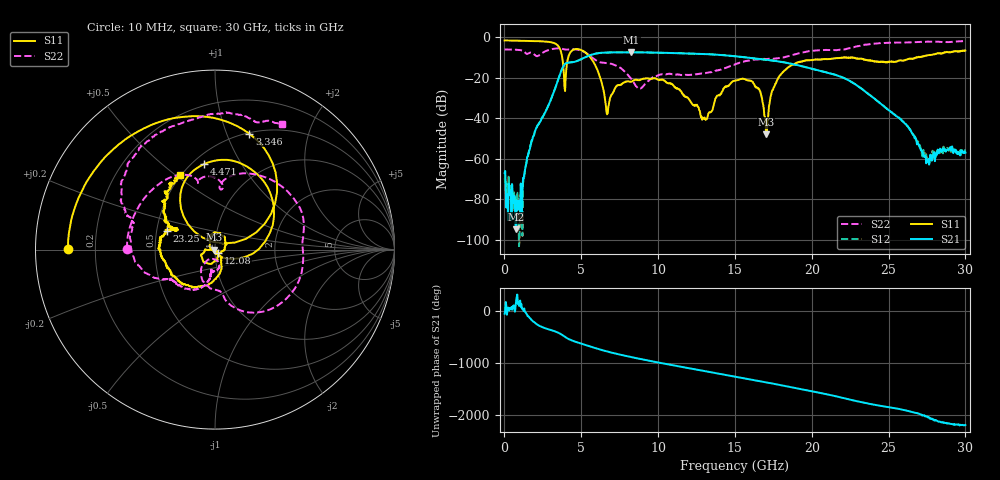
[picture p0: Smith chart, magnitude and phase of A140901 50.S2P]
!  2-Port S-parameters saved by WinCal
! VAR MeasName=S-Parameters (CALIBRATED_DATA) read from VNA (N5244A)
! VAR MeasDate=11/3/2014 9:35:49 AM
! VAR NAME=A140901 50
! VAR FILENAME=A140901 50.S2P
! VAR DATE=11/3/2014 9:35:50 AM
! VAR PHYS_PORTS=1,2
# Hz S RI R 50
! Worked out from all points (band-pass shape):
!   801 points, 10 MHz to 30 GHz, reference 50 ohm
!   highest |S21| = -7.53 dB at 8.257 GHz (marker M1); lowest = -94.8 dB at 759.8 MHz (marker M2)
!   |S21| within 3 dB of the highest: 5.107 GHz to 16.22 GHz (11.11 GHz wide, 104 % of centre)
!   lowest |S11| = -47.9 dB at 17.03 GHz (marker M3), VSWR 1.01, Z = 49.6 - j0.0285 ohm
!   |S11| at or under -10 dB: 3.756 GHz to 4.154 GHz (397.9 MHz wide, 10.1 % of centre); 5.58 GHz to 22.08 GHz (16.5 GHz wide, 119 % of centre); 22.1 GHz to 26.84 GHz (4.749 GHz wide, 19.4 % of centre)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
!   |S22| runs from -25.5 to -2.0 dB; largest |S21 - S12| = 0.0029
!   S11 on the Smith chart (normalised r, x): 10 MHz: 0.10, +0.00; 3.346 GHz: 0.51, +1.21; 4.471 GHz: 0.57, +0.70; 12.08 GHz: 1.03, -0.04; 23.25 GHz: 0.57, +0.13; 30 GHz: 0.49, +0.52
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1e7  -0.8175 0.00333  0.000247 -0.000369  0.000278 -0.000174  -0.4911 0.00373
7.5975e8  -0.7772 0.2442  -1.81e-05 -2.44e-06  2.49e-05 -3.71e-05  -0.3671 0.3175
1.921862e9  -0.5489 0.5745  -0.00304 0.00218  -0.00298 0.00225  0.0354 0.3725
3.346388e9  0.1907 0.6461  0.0441 -0.0413  0.0445 -0.0414  0.4163 0.3111
3.946188e9  -0.0154 0.0438  -0.1737 -0.13  -0.174 -0.1296  0.4878 0.0504
4.471012e9  -0.0615 0.4764  -0.1818 0.1566  -0.181 0.1564  0.4791 -0.1403
5.033325e9  0.2665 0.3866  0.0283 0.2868  0.0282 0.2863  0.3113 -0.3316
5.970512e9  0.1769 -0.0378  0.3899 -0.025  0.3897 -0.0242  0.048 -0.2599
6.682775e9  -0.00831 -0.00921  0.1857 -0.37  0.1858 -0.3693  0.00449 -0.2241
8.25725e9  -0.0194 0.0766  -0.4159 -0.0597  -0.4144 -0.0602  -0.0561 -0.0736
1.001916e10  0.0384 0.0793  0.0471 0.408  0.0469 0.4069  0.0118 -0.1132
1.208098e10  0.0165 -0.0209  0.3392 -0.194  0.3389 -0.1933  -0.0218 -0.1142
1.305565e10  -0.0016 -0.00934  0.0515 -0.3763  0.0504 -0.3754  -0.0247 -0.1251
1.5005e10  -0.0264 -0.0789  -0.3307 0.0491  -0.3299 0.0498  -0.0607 -0.2027
1.65045e10  -0.0529 -0.000149  -0.00313 0.2881  -0.00347 0.2885  -0.1895 -0.2063
1.702932e10  -0.00403 -0.000287  0.1285 0.2408  0.1271 0.2416  -0.2185 -0.1875
1.796651e10  0.0346 -0.1098  0.2414 0.0385  0.2416 0.0402  -0.2552 -0.1686
2.002832e10  -0.2217 -0.154  -0.0579 -0.153  -0.057 -0.1537  -0.4509 -0.048
2.325225e10  -0.2684 0.1054  0.0409 0.033  0.041 0.0332  -0.5194 0.3366
2.501416e10  -0.2104 0.1145  0.00881 -0.013  0.00887 -0.0129  -0.3338 0.6386
2.752582e10  -0.2847 0.2045  -0.000383 0.00076  -0.000426 0.000745  0.0536 0.7619
3e10  -0.1978 0.4158  0.00109 -0.000898  0.00112 -0.000867  0.3742 0.7016
